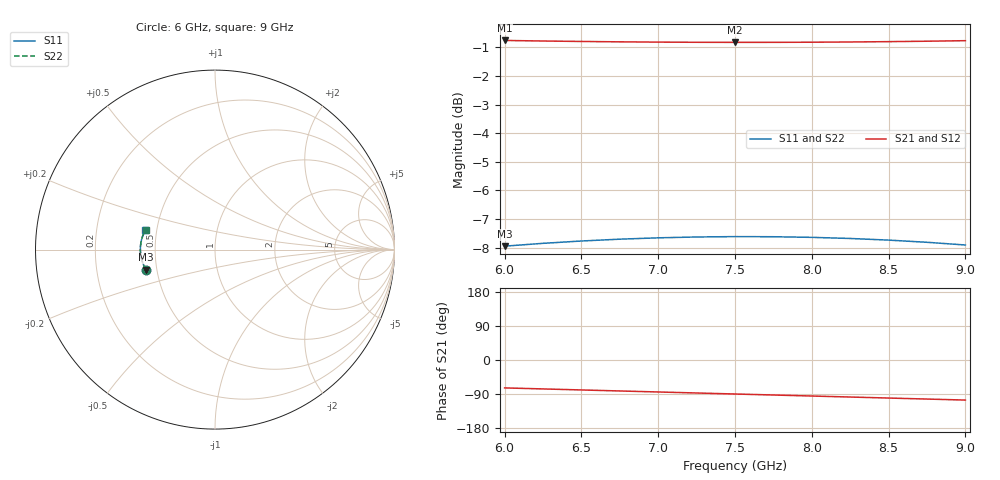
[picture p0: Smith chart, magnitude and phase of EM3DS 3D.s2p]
!AWR Design Environment (2469) Mon Oct 04 18:05:22 2004
!freq-unit  param-type  data-format  keyword  impedance-ohms
# GHz  S  MA  R  50
!Freq  MagS11  AngS11  MagS21  AngS21  MagS12  AngS12  MagS22  AngS22
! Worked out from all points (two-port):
!   13 points, 6 GHz to 9 GHz, reference 50 ohm
!   highest |S21| = -0.76 dB at 6 GHz (marker M1); lowest = -0.8 dB at 7.5 GHz (marker M2)
!   |S21| within 3 dB of the highest: start of sweep to end of sweep
!   lowest |S11| = -8.0 dB at 6 GHz (marker M3), VSWR 2.33, Z = 21.8 - j5.84 ohm
!   |S11| at or under -10 dB: nowhere
!   |S22| runs from -8.0 to -7.6 dB; largest |S21 - S12| = 0
6  0.4003 -163.7  0.9164 -73.6  0.9164 -73.6  0.4003 -163.6
6.25  0.4049 -166.3  0.9144 -76.3  0.9144 -76.3  0.4049 -166.3
6.5  0.4087 -169.0  0.9127 -79.0  0.9127 -79.0  0.4087 -169.0
6.75  0.4117 -171.7  0.9113 -81.7  0.9113 -81.7  0.4117 -171.7
7  0.4139 -174.4  0.9103 -84.4  0.9103 -84.4  0.4139 -174.4
7.25  0.4153 -177.0  0.9097 -87.1  0.9097 -87.1  0.4153 -177.1
7.5  0.416 -179.7  0.9094 -89.7  0.9094 -89.7  0.416 -179.8
7.75  0.4158 177.7  0.9095 -92.4  0.9095 -92.4  0.4158 177.5
8  0.4147 175.1  0.9099 -95.1  0.9099 -95.1  0.4147 174.8
8.25  0.4129 172.4  0.9108 -97.7  0.9108 -97.7  0.4129 172.1
8.5  0.4102 169.8  0.912 -100.4  0.912 -100.4  0.4102 169.4
8.75  0.4066 167.2  0.9136 -103.1  0.9136 -103.1  0.4066 166.7
9  0.4021 164.5  0.9156 -105.8  0.9156 -105.8  0.4021 164.0
